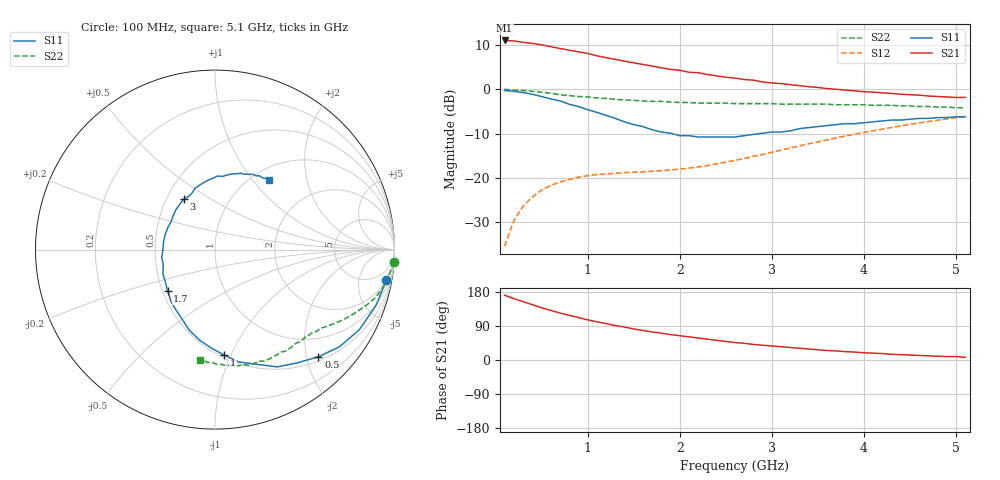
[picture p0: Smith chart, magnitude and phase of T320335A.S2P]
!AT-32033
!S PARAMETERS at Vce=5 V  Ic=1mA.  LAST UPDATED 01-05-95
# ghz s ma r 50
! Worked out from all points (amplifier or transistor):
!   51 points, 100 MHz to 5.1 GHz, reference 50 ohm
!   highest |S21| = 11.0 dB at 100 MHz (marker M1)
!   |S21| within 3 dB of that: start of sweep to 1.013 GHz
!   unconditionally stable (mu >= 1): 1.905 GHz to 2.741 GHz
!   at 900 MHz: K = 0.50, MSG = 14.1 dB, |S12| = -19.8 dB
!   at 2.6 GHz: K = 1.04, MAG = 8.0 dB, |S12| = -16.0 dB
!   at 5.1 GHz: K = 0.83, MSG = 2.2 dB, |S12| = -6.1 dB
!   S11 on the Smith chart (normalised r, x): 100 MHz: 2, -11; 500 MHz: 0.58, -2.23; 1 GHz: 0.52, -0.94; 1.7 GHz: 0.53, -0.28; 3 GHz: 0.61, +0.38; 5.1 GHz: 1.19, +1.21
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0.1  0.97 -10.0  3.56 171.0  0.017 84.0  1 -4.0
0.2  0.95 -19.0  3.52 162.0  0.033 78.0  0.98 -8.0
0.3  0.92 -29.0  3.39 154.0  0.048 72.0  0.97 -11.0
0.4  0.88 -38.0  3.3 146.0  0.061 68.0  0.95 -14.0
0.5  0.83 -46.0  3.18 138.0  0.073 63.0  0.93 -17.0
0.6  0.78 -54.0  3.03 131.0  0.082 59.0  0.9 -20.0
0.7  0.74 -62.0  2.89 124.0  0.09 55.0  0.87 -23.0
0.8  0.68 -70.0  2.77 118.0  0.096 53.0  0.85 -25.0
1  0.59 -85.0  2.54 106.0  0.106 49.0  0.82 -28.0
1.1  0.55 -92.0  2.39 101.0  0.109 47.0  0.8 -30.0
1.3  0.47 -108.0  2.18 91.0  0.113 45.0  0.77 -33.0
1.5  0.4 -123.0  1.99 82.0  0.116 45.0  0.75 -35.0
1.7  0.35 -139.0  1.83 74.0  0.119 47.0  0.73 -37.0
1.8  0.33 -147.0  1.75 71.0  0.121 48.0  0.73 -38.0
2  0.3 -164.0  1.64 64.0  0.126 51.0  0.71 -41.0
2.1  0.3 -172.0  1.56 61.0  0.129 53.0  0.71 -42.0
2.2  0.29 180.0  1.54 58.0  0.133 55.0  0.7 -43.0
2.6  0.29 148.0  1.34 46.0  0.158 61.0  0.69 -49.0
3  0.33 122.0  1.18 37.0  0.195 64.0  0.69 -55.0
3.5  0.38 99.0  1.05 27.0  0.256 64.0  0.68 -64.0
4.3  0.45 71.0  0.9 15.0  0.371 57.0  0.66 -80.0
5.1  0.49 52.0  0.81 7.0  0.493 45.0  0.62 -98.0
